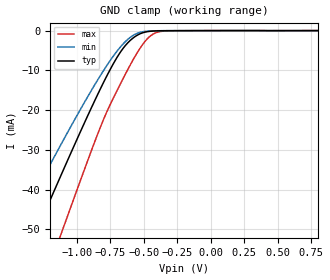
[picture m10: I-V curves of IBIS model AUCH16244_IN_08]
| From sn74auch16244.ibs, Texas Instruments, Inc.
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[Model]   AUCH16244_IN_08
Model_type  Input
Vinl=0.28
Vinh=0.52
| variable   typ   min   max
C_comp   3.37pF   2.67pF   3.91pF
[Temperature Range]   40   100   -40
| Ambient temperature   25   85   -40
[Voltage range]   0.8   0.8   0.8
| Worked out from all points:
|   GND clamp passes 1 mA (typ) near -0.54 V on its own axis
[GND Clamp]
| AUCH16244_IN_08
|   Voltage   I(typ)   I(min)   I(max)
-3.6V     -232.7mA   -194.4mA   -280.5mA
-1.465V   -63.19mA   -50.51mA   -83.5mA
-1.33V    -52.62mA   -41.83mA   -70.88mA
-1.285V   -49.12mA   -38.97mA   -66.67mA
-1.12V    -36.4mA    -28.63mA   -51.23mA
-1.085V   -33.73mA   -26.48mA   -47.96mA
-830mV    -14.98mA   -11.57mA   -24.69mA
-700mV    -6.699mA   -5.137mA   -15.04mA
-580mV    -1.847mA   -1.195mA   -7.304mA
-450mV    -162.3uA   -83.99uA   -1.323mA
-305mV    -21.19uA   -13.95uA   -49.01uA
800mV     109.4pA    199.4pA    88.89pA
